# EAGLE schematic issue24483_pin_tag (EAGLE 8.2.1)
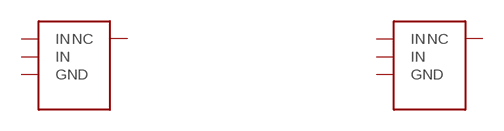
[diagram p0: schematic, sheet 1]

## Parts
U1  MYDEV  [DIP4]
U2  MYDEV_NC  (no package)
Unconnected: U1.1(IN) U1.2(IN) U1.4(NC) U2.GND U2.IN U2.NC

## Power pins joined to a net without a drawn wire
GND: U1.3(GND)

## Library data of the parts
U1 = tagtest:MYDEV
U2 = tagtest:MYDEV_NC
